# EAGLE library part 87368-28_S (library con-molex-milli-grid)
RECEPTACAL
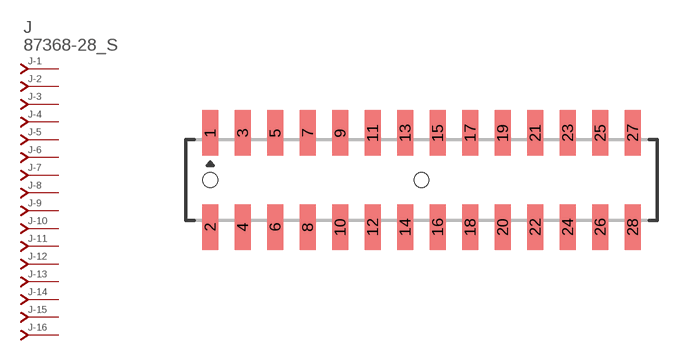
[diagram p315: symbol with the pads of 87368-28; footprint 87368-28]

Designator prefix J; gates -1=J-NV -2=J-N -3=J-N -4=J-N -5=J-N -6=J-N -7=J-N -8=J-N -9=J-N -10=J-N -11=J-N -12=J-N -13=J-N -14=J-N -15=J-N -16=J-N -17=J-N -18=J-N -19=J-N -20=J-N -21=J-N -22=J-N -23=J-N -24=J-N -25=J-N -26=J-N -27=J-N -28=J-N

## 87368-28_S  [87368-28]
1  -1:J  pas
2  -2:J  pas
3  -3:J  pas
4  -4:J  pas
5  -5:J  pas
6  -6:J  pas
7  -7:J  pas
8  -8:J  pas
9  -9:J  pas
10  -10:J  pas
11  -11:J  pas
12  -12:J  pas
13  -13:J  pas
14  -14:J  pas
15  -15:J  pas
16  -16:J  pas
17  -17:J  pas
18  -18:J  pas
19  -19:J  pas
20  -20:J  pas
21  -21:J  pas
22  -22:J  pas
23  -23:J  pas
24  -24:J  pas
25  -25:J  pas
26  -26:J  pas
27  -27:J  pas
28  -28:J  pas

## Footprint 87368-28 (pad centres in mm)
RECEPTACAL SMD Dual Row, Side Entry
smd 1 x 2.8: 1 -13,2.9; 2 -13,-2.9; 3 -11,2.9; 4 -11,-2.9; 5 -9,2.9; 6 -9,-2.9; 7 -7,2.9; 8 -7,-2.9; 9 -5,2.9; 10 -5,-2.9; 11 -3,2.9; 12 -3,-2.9; 13 -1,2.9; 14 -1,-2.9; 15 1,2.9; 16 1,-2.9; 17 3,2.9; 18 3,-2.9; 19 5,2.9; 20 5,-2.9; 21 7,2.9; 22 7,-2.9; 23 9,2.9; 24 9,-2.9; 25 11,2.9; 26 11,-2.9; 27 13,2.9; 28 13,-2.9
hole 0.914 at -13,0
hole 0.914 at 0,0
